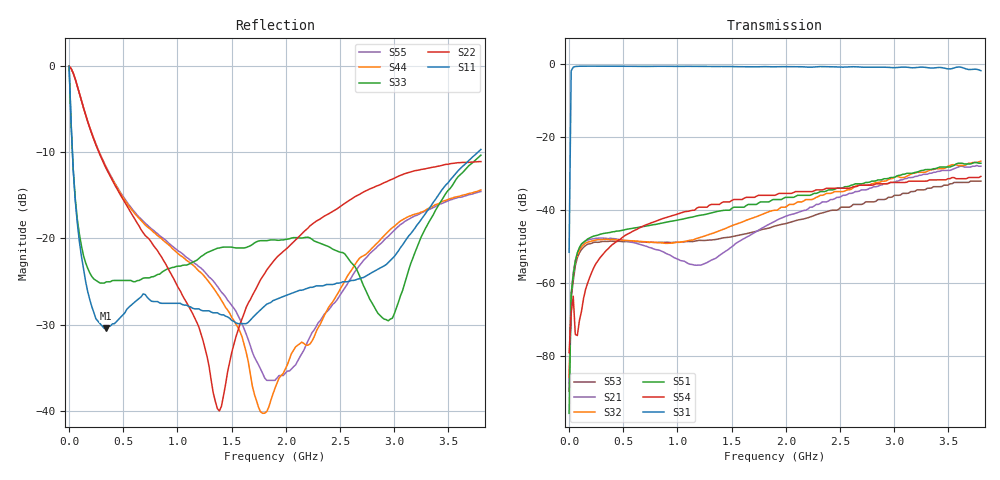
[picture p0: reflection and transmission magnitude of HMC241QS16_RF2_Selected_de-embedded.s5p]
! Hittite Microwave Corporation
! 20 Alpha Road
! Chelmsford, MA 01824
! Tel: 978-250-3343
! Fax: 978-250-3373
! Device: HMC241QS16, DC-3.5 GHz GaAs MMIC SP4T Non-Reflective Switch in 16 lead QSOP package
! Misc: Data was de-embedded to package pins.
!  Port 1 = RFC
!  Port 2 = RF1
!  Port 3 = RF2
!  Port 4 = RF3
!  Port 5 = RF4
!  Vdd  = + 5 V
!  RF2 selected, Vctl= 0/+5 V
!  Data reformated to new Touchstone file format - Tue Jan 09 10:07:35 2007
# MHz S DB R 50
! 5 Port Network Data
! freq  dbS11  angS11  dbS12  angS12  dbS13  angS13  dbS14  angS14
!  dbS15  angS15
!  dbS21  angS21  dbS22  angS22  dbS23  angS23
!  dbS24  angS24  dbS25  angS25
!  dbS31  angS31  dbS32  angS32
!  dbS33  angS33  dbS34  angS34  dbS35  angS35
!  dbS41  angS41
!  dbS42  angS42  dbS43  angS43  dbS44  angS44  dbS45  angS45
!  dbS51  angS51  dbS52  angS52  dbS53  angS53  dbS54  angS54
!  dbS55  angS55
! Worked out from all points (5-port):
!   201 points, 30 kHz to 3.8 GHz, reference 50 ohm
!   strongest paths, dB at 30 kHz, 950 MHz, 1.9 GHz, 2.85 GHz, 3.8 GHz:
!     S31: -51.5, -0.6, -0.7, -0.8, -1.8
!     S54: -79.0, -41.5, -35.9, -32.8, -30.8
!     S51: -95.6, -43.0, -37.1, -31.7, -27.1
!     S32: -85.8, -49.0, -40.0, -32.4, -26.6
!     S21: -87.5, -52.6, -43.0, -33.5, -28.0
!     S53: -89.6, -48.9, -44.3, -37.1, -32.0
!   lowest |S11| = -30.5 dB at 342 MHz (marker M1), VSWR 1.06, Z = 53 - j0.701 ohm
!   |S11| at or under -10 dB: 30.62 MHz to 3.772 GHz (3.741 GHz wide, 197 % of centre)
